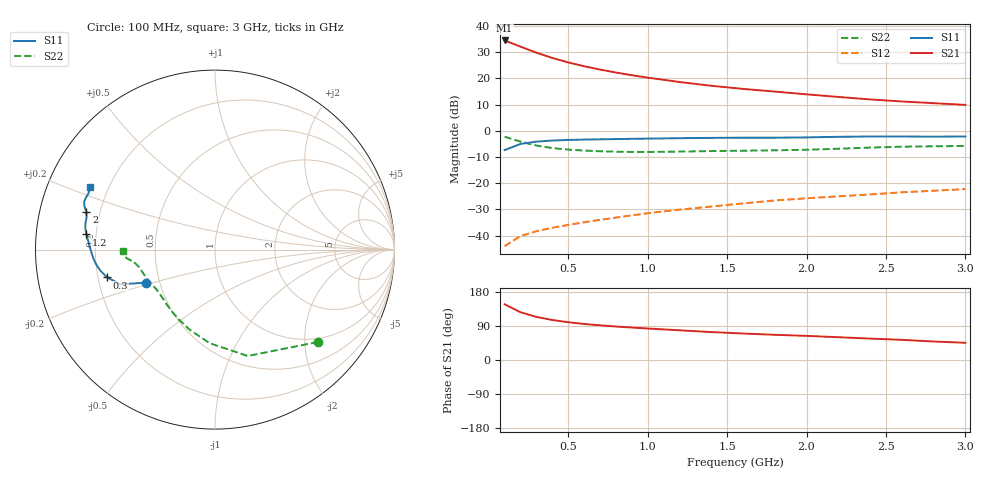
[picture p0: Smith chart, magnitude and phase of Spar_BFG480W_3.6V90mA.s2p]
! Filename: 3_690BFG480.001
! Title: BFG480W
! Bias: Vce=3.6V; Ic=90mA
! Company: NXP Semiconductors NL
! User: Quality&Reliability T&D
! Measure time: 10 Nov 1999 / 12:00:46
#  MHz  S  MA  R 50
! Freq  S11  S21  S12  S22  :
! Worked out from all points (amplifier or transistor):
!   20 points, 100 MHz to 3 GHz, reference 50 ohm
!   highest |S21| = 34.5 dB at 100 MHz (marker M1)
!   |S21| within 3 dB of that: start of sweep to 227.6 MHz
!   unconditionally stable (mu >= 1): 746.9 MHz to end of sweep
!   at 400 MHz: K = 0.79, MSG = 32.4 dB, |S12| = -37.0 dB
!   at 1.2 GHz: K = 1.07, MAG = 22.7 dB, |S12| = -30.1 dB
!   at 3 GHz: K = 1.05, MAG = 14.7 dB, |S12| = -22.3 dB
!   S11 on the Smith chart (normalised r, x): 100 MHz: 0.42, -0.19; 300 MHz: 0.24, -0.12; 1.2 GHz: 0.16, +0.06; 2 GHz: 0.15, +0.14; 3 GHz: 0.13, +0.23
100  0.4273 -154.5  52.79 147.1  0.00628 69.3  0.771 -41.9
200  0.5609 -159.8  40.24 126.0  0.009808 60.3  0.62 -72.9
300  0.62 -165.5  30.8 113.7  0.0121 59.1  0.5218 -93.4
400  0.6499 -169.7  24.47 105.6  0.01408 60.5  0.4677 -107.6
500  0.6675 -173.0  20.17 99.7  0.01598 62.6  0.4371 -117.9
600  0.6786 -175.6  17.03 95.1  0.0179 64.4  0.4187 -125.6
700  0.6862 -177.9  14.72 91.5  0.01997 66.4  0.4064 -131.6
800  0.6929 180.0  12.91 88.3  0.02205 68.2  0.3986 -136.6
900  0.7008 178.1  11.47 85.7  0.02429 70.0  0.3945 -140.9
1000  0.7072 176.3  10.31 83.1  0.02666 71.1  0.3938 -144.7
1200  0.7212 173.3  8.515 78.4  0.03122 72.7  0.4001 -150.9
1400  0.7312 171.0  7.208 73.7  0.0358 73.8  0.4098 -155.5
1600  0.7367 168.6  6.288 69.9  0.04107 74.6  0.4158 -159.0
1800  0.7371 166.0  5.591 66.5  0.04676 75.1  0.423 -162.7
2000  0.7466 163.8  4.949 63.6  0.05145 75.9  0.4341 -167.1
2200  0.7664 161.6  4.417 60.1  0.056 75.7  0.4534 -170.7
2400  0.7762 159.9  3.96 56.5  0.06089 75.2  0.4775 -173.1
2600  0.7754 158.2  3.621 53.2  0.06695 74.5  0.496 -174.5
2800  0.7715 156.0  3.357 48.8  0.07172 73.2  0.505 -176.3
3000  0.7764 153.3  3.117 45.4  0.07706 72.4  0.5124 -179.2
